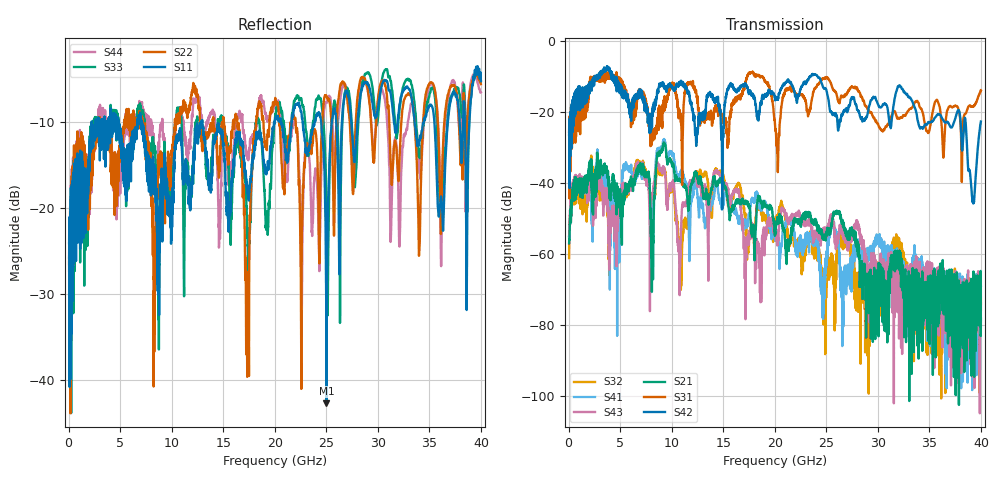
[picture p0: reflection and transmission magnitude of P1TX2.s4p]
!Agilent Technologies,N5245A,MY49151084,A.09.20.08
!Agilent N5245A: A.09.20.08
!Date: Thursday, March 01, 2012 14:43:28
!Correction: S11(Full 4 Port(1,2,3,4))
!S12(Full 4 Port(1,2,3,4))
!S13(Full 4 Port(1,2,3,4))
!S14(Full 4 Port(1,2,3,4))
!S21(Full 4 Port(1,2,3,4))
!S22(Full 4 Port(1,2,3,4))
!S23(Full 4 Port(1,2,3,4))
!S24(Full 4 Port(1,2,3,4))
!S31(Full 4 Port(1,2,3,4))
!S32(Full 4 Port(1,2,3,4))
!S33(Full 4 Port(1,2,3,4))
!S34(Full 4 Port(1,2,3,4))
!S41(Full 4 Port(1,2,3,4))
!S42(Full 4 Port(1,2,3,4))
!S43(Full 4 Port(1,2,3,4))
!S44(Full 4 Port(1,2,3,4))
!S4P File: Measurements: <S11,S12,S13,S14>,
!<S21,S22,S23,S24>,
!<S31,S32,S33,S34>,
!<S41,S42,S43,S44>:
# Hz S  dB  R 50
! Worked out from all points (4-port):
!   3996 points, 50 MHz to 40 GHz, reference 50 ohm
!   strongest paths, dB at 50 MHz, 10.04 GHz, 20.03 GHz, 30.02 GHz, 40 GHz:
!     S42: -26.4, -12.9, -16.5, -17.8, -22.7
!     S31: -25.5, -12.1, -23.7, -23.3, -13.9
!     S21: -57.0, -34.9, -53.8, -72.7, -78.2
!     S43: -55.3, -40.4, -52.2, -67.4, -75.7
!     S41: -55.1, -32.0, -54.4, -56.2, -69.0
!     S32: -61.2, -41.9, -50.5, -73.8, -74.1
!   lowest |S11| = -42.7 dB at 25.02 GHz (marker M1), VSWR 1.01, Z = 50.3 - j0.683 ohm
!   |S11| at or under -10 dB: start of sweep to 2.239 GHz; 7.12 GHz to 12.87 GHz (5.747 GHz wide, 57.5 % of centre); 12.97 GHz to 20 GHz (7.026 GHz wide, 42.6 % of centre)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
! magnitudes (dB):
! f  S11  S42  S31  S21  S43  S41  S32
! 50 MHz  -24.1  -26.4  -25.5  -57.0  -55.3  -55.1  -61.2
! 8.11 GHz  -17.5  -19.1  -26.0  -53.3  -43.4  -54.0  -50.2
! 9.23 GHz  -17.4  -12.7  -17.1  -29.1  -35.9  -27.8  -36.6
! 10.83 GHz  -11.0  -12.1  -20.8  -39.1  -59.0  -37.1  -58.6
! 14.34 GHz  -11.3  -16.0  -18.8  -40.5  -36.4  -40.1  -36.2
! 25.02 GHz  -42.7  -13.9  -10.1  -54.2  -55.3  -61.3  -66.2
! 40 GHz  -5.3  -22.7  -13.9  -78.2  -75.7  -69.0  -74.1
